{attribute 'qualified_only'}
TYPE E_FunctionType :
(
	Sine,		// typical for vibrations originating from rotating machine
	Square,		// mixed sine signals good for analyzing spectrum
	Pulse,		// mixed sine signals good for analyzing spectrum
	Triangular,	// mixed sine signals good for analyzing spectrum
	Sawtooth,	// ramp-type vibrations, continuously increasing
	AM,			// amplitude modulation: typical for vibrations originating from gear-tooth failure or bearing faults
	Harmonics,	// summed up sine signals good for analyzing cepstrum
	Shock,		// shock with exponential decay
	Shockwave	// shockwave (sine) with exponential decay
);
END_TYPE
